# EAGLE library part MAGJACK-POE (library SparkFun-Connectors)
PoE compatible MagJack This is a simple RJ45 PoEthernet MagJack connector that can help connect you to the Internet with the ability to provide power. Here is the connector we sell at SparkFun: RJ45 PoE MagJack (PRT-13606) Note: This connector is not on any currently live SparkFun products, however it has been used on previously reitred products, so the package is proven.
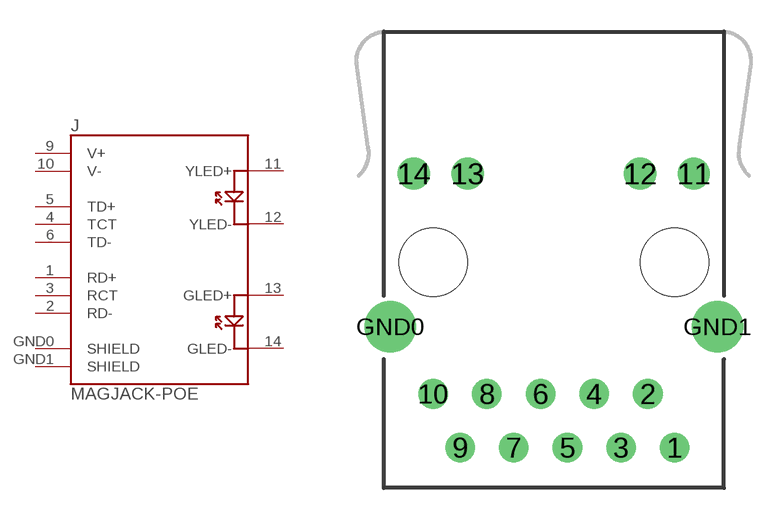
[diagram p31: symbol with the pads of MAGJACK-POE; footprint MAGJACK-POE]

Designator prefix J

## MAGJACK-POE (PROD_ID: CONN-10659; SF_ID: PRT-13606)  [MAGJACK-POE]
1  RD+
2  RD-
3  RCT
4  TCT
5  TD+
6  TD-
9  V+
10  V-
11  YLED+
12  YLED-
13  GLED+
14  GLED-
GND0  SHIELD
GND1  SHIELD

## Footprint MAGJACK-POE (pad centres in mm)
RJ45 PoE MagJack This RJ-45 jack with magnetics, gives you access to the unused twisted pair (10BASE-T, and 100BASE-T) which usually carries power in a power-over-ethernet system. Specifications: Pin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
drill 0.89: 1 5.72,-8.89; 2 4.45,-6.35; 3 3.18,-8.89; 4 1.91,-6.35; 5 0.64,-8.89; 6 -0.63,-6.35; 7 -1.9,-8.89; 8 -3.17,-6.35; 9 -4.44,-8.89; 10 -5.71,-6.35
drill 1.02: 11 6.625,4.08; 12 4.085,4.08; 13 -4.085,4.08; 14 -6.625,4.08
drill 1.63: GND0 -7.745,-3.17; GND1 7.745,-3.17
hole 3.25 at -5.715,-0.12
hole 3.25 at 5.715,-0.12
